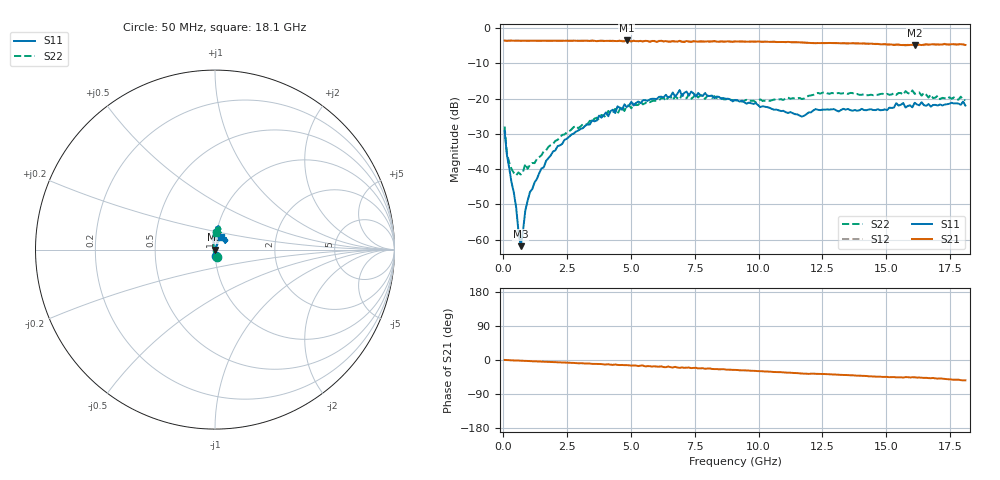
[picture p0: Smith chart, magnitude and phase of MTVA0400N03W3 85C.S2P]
! Network Analyzer HP8720D.06.14 Serial No. US36140669
!  7 Jul 2005  13:45:42
! Frequency  S11  S21  S12  S22
# HZ  S  DB R 50
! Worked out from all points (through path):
!   201 points, 50 MHz to 18.1 GHz, reference 50 ohm
!   highest |S21| = -3.49 dB at 4.833 GHz (marker M1); lowest = -4.8 dB at 16.11 GHz (marker M2)
!   group delay of S21, straight-line fit = 8.21 ps
!   lowest |S11| = -61.9 dB at 681.8 MHz (marker M3), VSWR 1.00, Z = 49.9 + j0.00173 ohm
!   |S11| at or under -10 dB: start of sweep to end of sweep
!   |S22| runs from -41.8 to -17.7 dB; largest |S21 - S12| = 0.024
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5e7  -29.25 -82.2  -3.54 0.2  -3.54 0.1  -27.92 -76.8
1.4025e8  -35.96 -84.9  -3.59 -0.2  -3.58 -0.3  -35.50 -109.1
2.305e8  -39.71 -87.1  -3.56 -0.6  -3.55 -0.6  -38.13 -125.8
5.0125e8  -50.82 -96.7  -3.57 -1.5  -3.56 -1.5  -41.77 -169.2
6.8175e8  -61.85 178.8  -3.56 -1.9  -3.57 -2.0  -41.52 172.8
8.6225e8  -51.68 80.0  -3.56 -2.3  -3.57 -2.4  -38.50 161.7
1.04275e9  -46.50 86.0  -3.56 -3.0  -3.55 -3.0  -38.77 141.0
1.494e9  -39.77 76.6  -3.58 -4.2  -3.57 -4.3  -36.07 121.6
2.12575e9  -33.47 67.5  -3.57 -6.1  -3.57 -6.1  -31.70 107.0
3.1185e9  -28.36 71.3  -3.59 -8.6  -3.62 -9.0  -27.26 105.6
4.382e9  -24.10 71.6  -3.66 -11.9  -3.63 -12.9  -22.90 97.0
4.47225e9  -22.19 68.7  -3.67 -12.9  -3.59 -12.3  -24.29 99.6
4.83325e9  -22.39 78.2  -3.49 -13.6  -3.60 -14.4  -22.02 87.6
6.09675e9  -19.50 76.5  -3.67 -17.6  -3.59 -17.6  -20.44 85.8
6.909e9  -17.56 82.5  -3.59 -20.7  -3.70 -19.7  -20.23 79.0
7.54075e9  -19.45 79.7  -3.77 -20.4  -3.63 -22.3  -18.54 85.1
9.075e9  -20.37 92.3  -3.79 -26.1  -3.77 -26.2  -20.45 77.2
1.169225e10  -25.09 81.7  -4.08 -35.7  -4.07 -35.6  -20.11 78.4
1.21435e10  -23.35 79.9  -4.25 -36.0  -4.20 -36.2  -18.93 80.8
1.512175e10  -22.57 37.9  -4.67 -45.4  -4.55 -45.1  -18.92 85.6
1.61145e10  -21.18 43.5  -4.84 -45.6  -4.62 -45.9  -18.63 81.4
1.81e10  -21.95 63.7  -4.77 -53.6  -4.86 -54.5  -20.43 87.4
